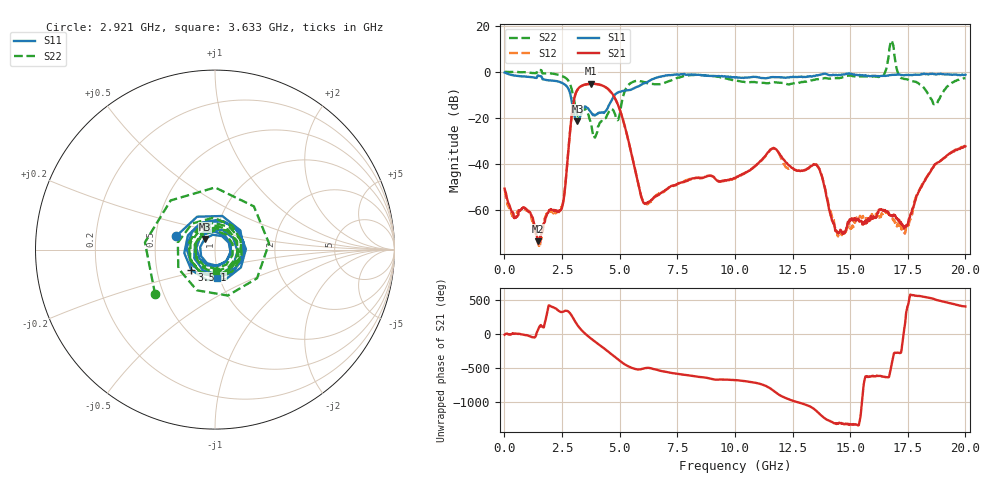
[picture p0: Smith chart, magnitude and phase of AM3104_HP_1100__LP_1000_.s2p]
!Created with skrf (http://scikit-rf.org).
# Hz S RI R 50.0
!freq ReS11 ImS11 ReS21 ImS21 ReS12 ImS12 ReS22 ImS22
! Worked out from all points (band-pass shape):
!   1601 points, 10 MHz to 20 GHz, reference 50 ohm
!   highest |S21| = -5.17 dB at 3.746 GHz (marker M1); lowest = -73.8 dB at 1.447 GHz (marker M2)
!   |S21| within 3 dB of the highest: 3.151 GHz to 4.565 GHz (1.414 GHz wide, 36.6 % of centre)
!   lowest |S11| = -21.6 dB at 3.171 GHz (marker M3), VSWR 1.18, Z = 44.2 + j5.28 ohm
!   |S11| at or under -10 dB: 2.865 GHz to 4.796 GHz (1.931 GHz wide, 50.4 % of centre)
!   |S22| runs from -28.7 to 13.6 dB; largest |S21 - S12| = 0.042
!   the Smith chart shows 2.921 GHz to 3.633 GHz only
!   S11 on the Smith chart (normalised r, x): 2.921 GHz: 0.64, +0.10; 3.521 GHz: 0.75, -0.18; 3.633 GHz: 0.97, -0.32
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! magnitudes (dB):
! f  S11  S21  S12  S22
! 10 MHz  -0.4  -50.9  -51.5  -0.1
! 1.447 GHz  -1.6  -73.8  -73.5  0.8
! 2.509 GHz  -4.9  -58.8  -58.3  -1.9
! 2.921 GHz  -12.8  -18.9  -19.0  -7.6
! 3.171 GHz  -21.6  -7.8  -7.9  -19.1
! 3.346 GHz  -18.0  -6.2  -6.2  -17.8
! 3.521 GHz  -15.2  -5.6  -5.6  -16.4
! 3.633 GHz  -16.0  -5.3  -5.4  -18.4
! 3.746 GHz  -17.5  -5.2  -5.2  -22.3
! 4.883 GHz  -9.2  -13.3  -13.3  -20.8
! 5.345 GHz  -8.1  -28.5  -28.4  -6.2
! 6.032 GHz  -5.1  -57.0  -56.8  -4.4
! 6.682 GHz  -2.4  -53.6  -53.2  -5.5
! 10.01 GHz  -2.5  -46.3  -46.5  -3.9
! 11.64 GHz  -2.4  -33.4  -33.4  -4.5
! 13.34 GHz  -2.1  -41.0  -40.8  -3.8
! 14.54 GHz  -1.4  -69.8  -70.9  -2.8
! 16.38 GHz  -1.8  -60.2  -61.8  -2.2
! 16.68 GHz  -1.6  -61.9  -62.0  7.2
! 17.41 GHz  -1.4  -67.4  -68.5  -3.2
! 18.68 GHz  -1.0  -40.4  -40.5  -14.0
! 20 GHz  -1.3  -32.5  -32.2  -2.8
